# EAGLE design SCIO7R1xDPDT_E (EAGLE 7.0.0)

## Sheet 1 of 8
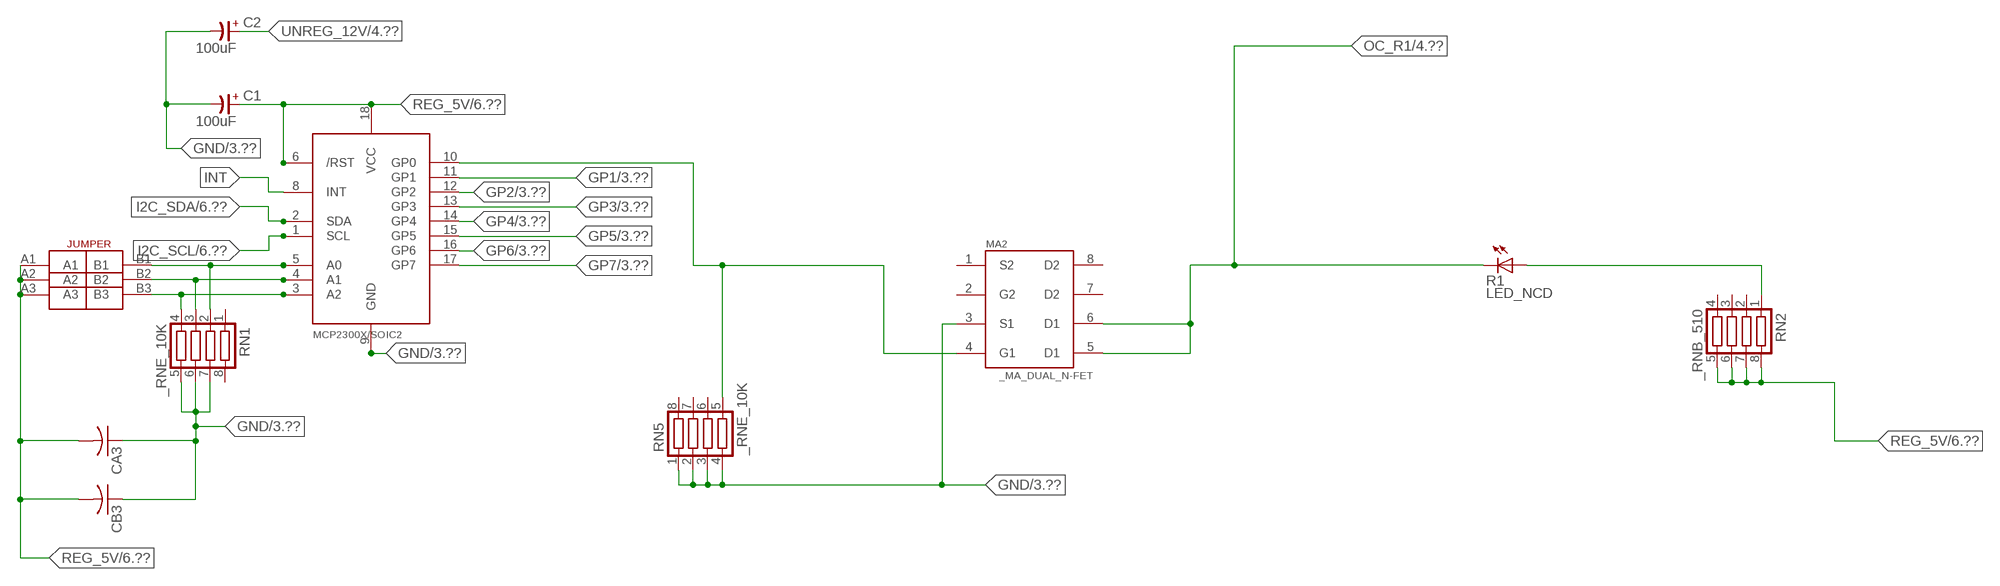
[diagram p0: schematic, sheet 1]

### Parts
C1  100uF  CP-E-025X060  [E-025X060]
C2  100uF  CP-E-025X060  [E-025X060]
CA3  CC1206KRX7R9BB104C1206K  [CC1206KRX7R9BB104]
CB3  TMK316F106ZL-TC1206K  [TMK316F106ZL-T]
IC2  MCP2300X/SO  [SO18W]
MA2  _MA_DUAL_N-FET  [_MA_DUAL_N-FET]
R1  LED_NCD  [CHIPLED_0603]
RN1  _RNE_10K  [RNE]
RN2  _RNB_510  [RNB]
RN5  _RNE_10K  [RNE]
U$18  JUMPER_3X2  [JUMPER_3X2]

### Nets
GND: C1.- C2.- CA3.1 CB3.1 IC2.9(GND) MA2.3(S1) RN1.5 RN1.6 RN1.7 RN5.1 RN5.2 RN5.3 RN5.4 ; also sheet 3,6,8
GP1: IC2.11(GP1) ; also sheet 3
GP2: IC2.12(GP2) ; also sheet 3
GP3: IC2.13(GP3) ; also sheet 3
GP4: IC2.14(GP4) ; also sheet 3
GP5: IC2.15(GP5) ; also sheet 3
GP6: IC2.16(GP6) ; also sheet 3
GP7: IC2.17(GP7) ; also sheet 3
I2C_SCL: IC2.1(SCL) ; also sheet 6
I2C_SDA: IC2.2(SDA) ; also sheet 6
INT: IC2.8(INT)
N$6: IC2.5(A0) RN1.2 U$18.B1
N$7: IC2.4(A1) RN1.3 U$18.B2
N$8: IC2.3(A2) RN1.4 U$18.B3
N$23: IC2.10(GP0) MA2.4(G1) RN5.5
N$32: R1.A RN2.1
OC_R1: MA2.5(D1) MA2.6(D1) R1.C ; also sheet 4
REG_5V: C1.+ CA3.2 CB3.2 IC2.6(/RST) IC2.18(VCC) RN2.5 RN2.6 RN2.7 RN2.8 U$18.A1 U$18.A2 U$18.A3 ; also sheet 6,8
UNREG_12V: C2.+ ; also sheet 4,6
Unconnected: MA2.2(G2) MA2.7(D2) MA2.8(D2) RN1.1 RN1.8 RN2.2 RN2.3 RN2.4 RN5.6 RN5.7 RN5.8

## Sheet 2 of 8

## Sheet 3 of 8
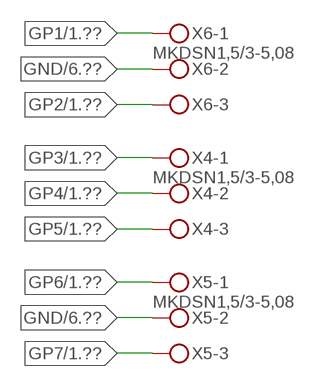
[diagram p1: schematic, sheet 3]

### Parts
X4  MKDSN1,5/3-5,08  [MKDSN1,5/3-5,08]
X5  MKDSN1,5/3-5,08  [MKDSN1,5/3-5,08]
X6  MKDSN1,5/3-5,08  [MKDSN1,5/3-5,08]

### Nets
GND: X5.2 X6.2 ; also sheet 1,6,8
GP1: X6.1 ; also sheet 1
GP2: X6.3 ; also sheet 1
GP3: X4.1 ; also sheet 1
GP4: X4.2 ; also sheet 1
GP5: X4.3 ; also sheet 1
GP6: X5.1 ; also sheet 1
GP7: X5.3 ; also sheet 1

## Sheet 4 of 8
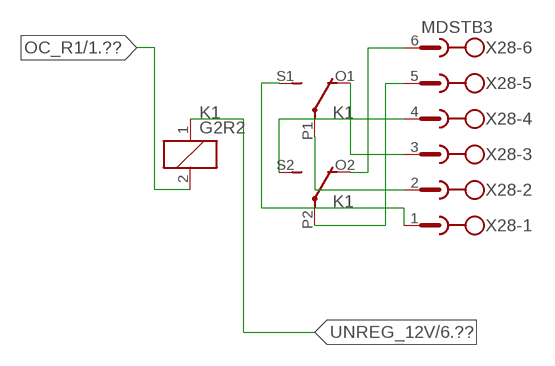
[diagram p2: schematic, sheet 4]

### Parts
K1  G2R2  [G2R2]
X28  MDSTB3  [MDSTB3]

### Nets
N$203: K1.P2(3:COM) X28.5
N$204: K1.O2(3:NC) X28.6
N$205: K1.S2(3:NO) X28.4
N$206: K1.P1(2:COM) X28.2
N$207: K1.O1(2:NC) X28.3
N$208: K1.S1(2:NO) X28.1
OC_R1: K1.2(1:C2) ; also sheet 1
UNREG_12V: K1.1(1:C1) ; also sheet 1,6

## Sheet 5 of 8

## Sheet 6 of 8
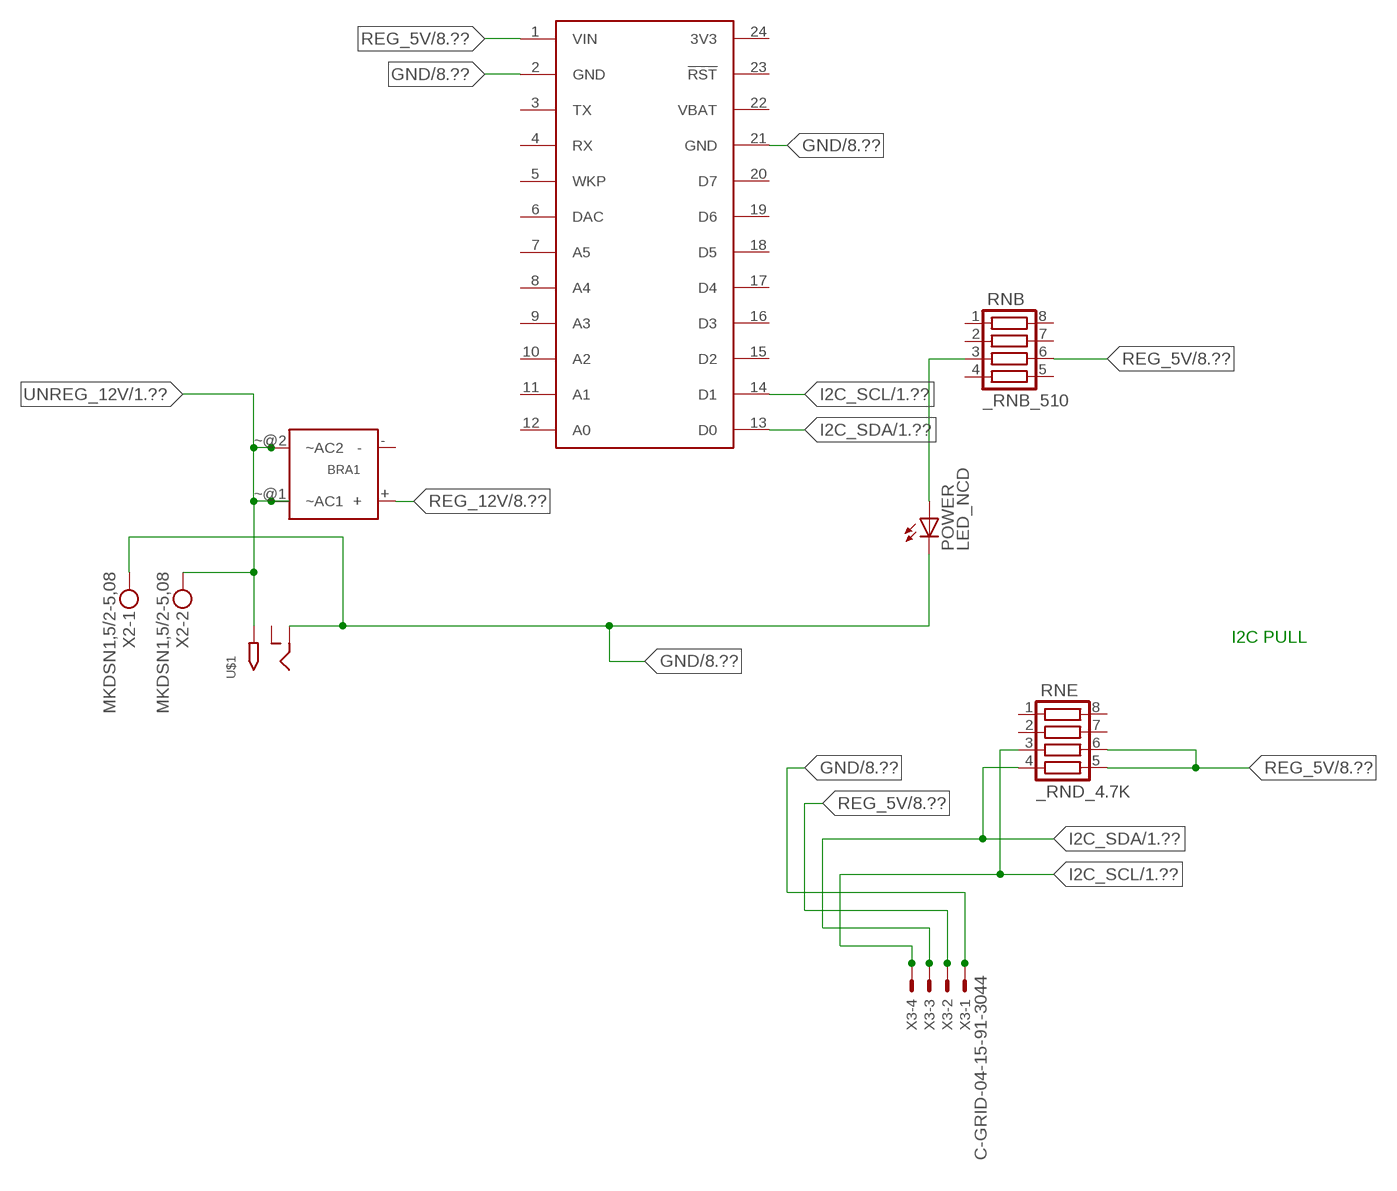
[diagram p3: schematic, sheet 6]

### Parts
BRA1  MB2S_  [MB2S]
POWER  LED_NCD  [CHIPLED_0603]
RNB  _RNB_510  [RNB]
RNE  _RND_4.7K  [RND]
S1  SPARK_CORECORE  [SPARK_CORE]
U$1  2.1MMJACK  [PJ-102A]
X2  MKDSN1,5/2-5,08  [MKDSN1,5/2-5,08]
X3  C-GRID-04-15-91-3044  [15-91-04]

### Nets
GND: POWER.C S1.2(GND) S1.21(GND) U$1.RING X2.1 X3.1 ; also sheet 1,3,8
I2C_SCL: RNE.3 S1.14(D1) X3.4 ; also sheet 1
I2C_SDA: RNE.4 S1.13(D0) X3.3 ; also sheet 1
N$2: POWER.A RNB.3
REG_5V: RNB.6 RNE.5 RNE.6 S1.1(VIN) X3.2 ; also sheet 1,8
REG_12V: BRA1.+ ; also sheet 8
UNREG_12V: BRA1.~@1(~AC1) BRA1.~@2(~AC2) U$1.TIP X2.2 ; also sheet 1,4
Unconnected: BRA1.- RNB.1 RNB.2 RNB.4 RNB.5 RNB.7 RNB.8 RNE.1 RNE.2 RNE.7 RNE.8 S1.3(TX) S1.4(RX) S1.5(WKP) S1.6(DAC) S1.7(A5) S1.8(A4) S1.9(A3) S1.10(A2) S1.11(A1) S1.12(A0) S1.15(D2) S1.16(D3) S1.17(D4) S1.18(D5) S1.19(D6) S1.20(D7) S1.23(!RST) U$1.RING_SW

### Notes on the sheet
- I2C PULL

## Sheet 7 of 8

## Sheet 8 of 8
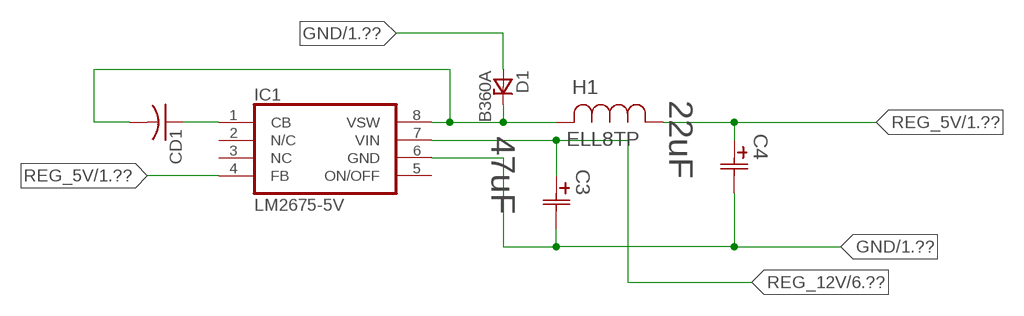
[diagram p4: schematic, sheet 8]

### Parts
C3  47uF  490-5463-6-NDCAP  [C2917(7343)-Y]
C4  22uF  490-5463-6-NDCAP  [C2917(7343)-Y]
CD1  _CD_10NF_50VC1206K  [_CD_10NF_50V]
D1  B360A  [DO214AC_ZENER]
H1  ELL8TP  [IND_ELL8TP]
IC1  LM2675-5V  LM2675  [SO-8]

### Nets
GND: C3.2(C2) C4.2(C2) D1.A IC1.6(GND) ; also sheet 1,3,6
N$1: CD1.2 D1.C H1.2 IC1.8(VSW)
N$3: CD1.1 IC1.1(CB)
REG_5V: C4.1(C1) H1.1 IC1.4(FB) ; also sheet 1,6
REG_12V: C3.1(C1) IC1.7(VIN) ; also sheet 6
Unconnected: IC1.2(N/C) IC1.5(ON/OFF)

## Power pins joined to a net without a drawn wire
3V3: S1.24(3V3)
NC: IC1.3(NC)
S2: MA2.1(S2)
VBAT: S1.22(VBAT)

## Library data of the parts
BRA1 = NCD_ULTIMATE_LIBRARY:MB2S: Bridge Rectifier BRA MB2S 200V 500ma Digikey MB2S-TPMSTR-ND/MB2S-TP
C1 C2 = NCD_ULTIMATE_LIBRARY:CP-: Capacitors All Kinds POLARIZED CAP
C3 C4 = NCD_ULTIMATE_bhaskar:490-5463-6-ND: NCD CAP
CA3 = NCD_ULTIMATE_LIBRARY:CC1206KRX7R9BB104: Capacitor CA .1uF 50V SMT C1206K CC1206KRX7R9BB104
CB3 = NCD_ULTIMATE_LIBRARY:TMK316F106ZL-T: Capacitor CB 10uF SMT 1206 TMK316F106ZL-T
CD1 = NCD_ULTIMATE_LIBRARY:_CD_10NF_50V: Capacitor 10nF SMT
D1 = NCD_ULTIMATE_bhaskar:B360A: NCD DIODE B350A/B360A
H1 = NCD_ULTIMATE_bhaskar:ELL8TP: NCD coil
IC1 = NCD_ULTIMATE_bhaskar:LM2675: LM2675 NCD http://www.ti.com/lit/ds/symlink/lm2675.pdf
IC2 = NCD_ULTIMATE_LIBRARY:MCP2300X: Semiconductor Port Expander I/O 8-Bit I2C MCP23008 Inexpensive i2c i/o expander - 8 general purpose i/o pins with optional pullups
K1 = NCD_ULTIMATE_LIBRARY:G2R2: RELAY 2 x switch, Omron
MA2 = NCD_ULTIMATE_LIBRARY:_MA_DUAL_N-FET: FET Dual N-Channel 8-SOIC NMOSFET Digikey 785-1064-2-ND/AO4842
POWER = NCD_ULTIMATE_bhaskar:LED_NCD
R1 = NCD_ULTIMATE_LIBRARY:LED_NCD: LED Digikey 754-1132-2-ND/APT2012SRCPRV
RN1 RN5 = NCD_ULTIMATE_LIBRARY:_RNE_10K: Resistor Array RNE SMT 10K x 4 Single Resistor Source: http://www.ctscorp.com/components/Datasheets/CTSChipArrayDs.pdf Digikey 742C083103JPTR-ND/742C083103JP; OC_FARNELL: unknown; OC_NEWARK: unknown
RN2 RNB = NCD_ULTIMATE_LIBRARY:_RNB_510: Resistor Array RNB SMT 510 x 4 Single Resistor Source: http://www.ctscorp.com/components/Datasheets/CTSChipArrayDs.pdf Digikey 742C083511JPTR-ND/ 742C083511JP; OC_FARNELL: unknown; OC_NEWARK: unknown
RNE = NCD_ULTIMATE_LIBRARY:_RND_4.7K: Resistor Array RND SMT 4.7K x 4 Single Resistor Source: http://www.ctscorp.com/components/Datasheets/CTSChipArrayDs.pdf Digikey 742C083472JPTR-ND/742C083472JP; OC_FARNELL: unknown; OC_NEWARK: unknown
S1 = Spark:SPARK_CORE
U$1 = NCD_ULTIMATE_CONNECTORS:2.1MMJACK: 2.1mm x 5.5mm DC jack with internal switch. Digikey part #PJ-102A, 4UCON part #05537 By microbuilder.eu
U$18 = NCD_ULTIMATE_CONNECTORS:JUMPER_3X2
X2 = NCD_ULTIMATE_CONNECTORS:MKDSN1,5/2-5,08: MKDSN 1,5/ 2-5,08 Printklemme
X3 = NCD_ULTIMATE_CONNECTORS:C-GRID-04: CONNECTOR 4-Pos I2C wire to board 2.54 mm (0.100") pitch header Digikey WM1342-ND/0015912045; OC_FARNELL: unknown; OC_NEWARK: unknown
X4-X6 = NCD_ULTIMATE_CONNECTORS:MKDSN1,5/3-5,08: MKDSN 1,5/ 3-5,08 Printklemme Nennstrom: 13,5 A Nennspannung: 250 V Rastermaß: 5,08 mm Polzahl: 3 Anschlussart: Schraubanschluss Montage: Löten Anschlussrichtung Leiter/Platine: 0 ° Artikelnummer: 1729131 Source: http://eshop.phoenixcontact.com .. 1729131.pdf
X28 = NCD_ULTIMATE_LIBRARY:MDSTB3: PHOENIX

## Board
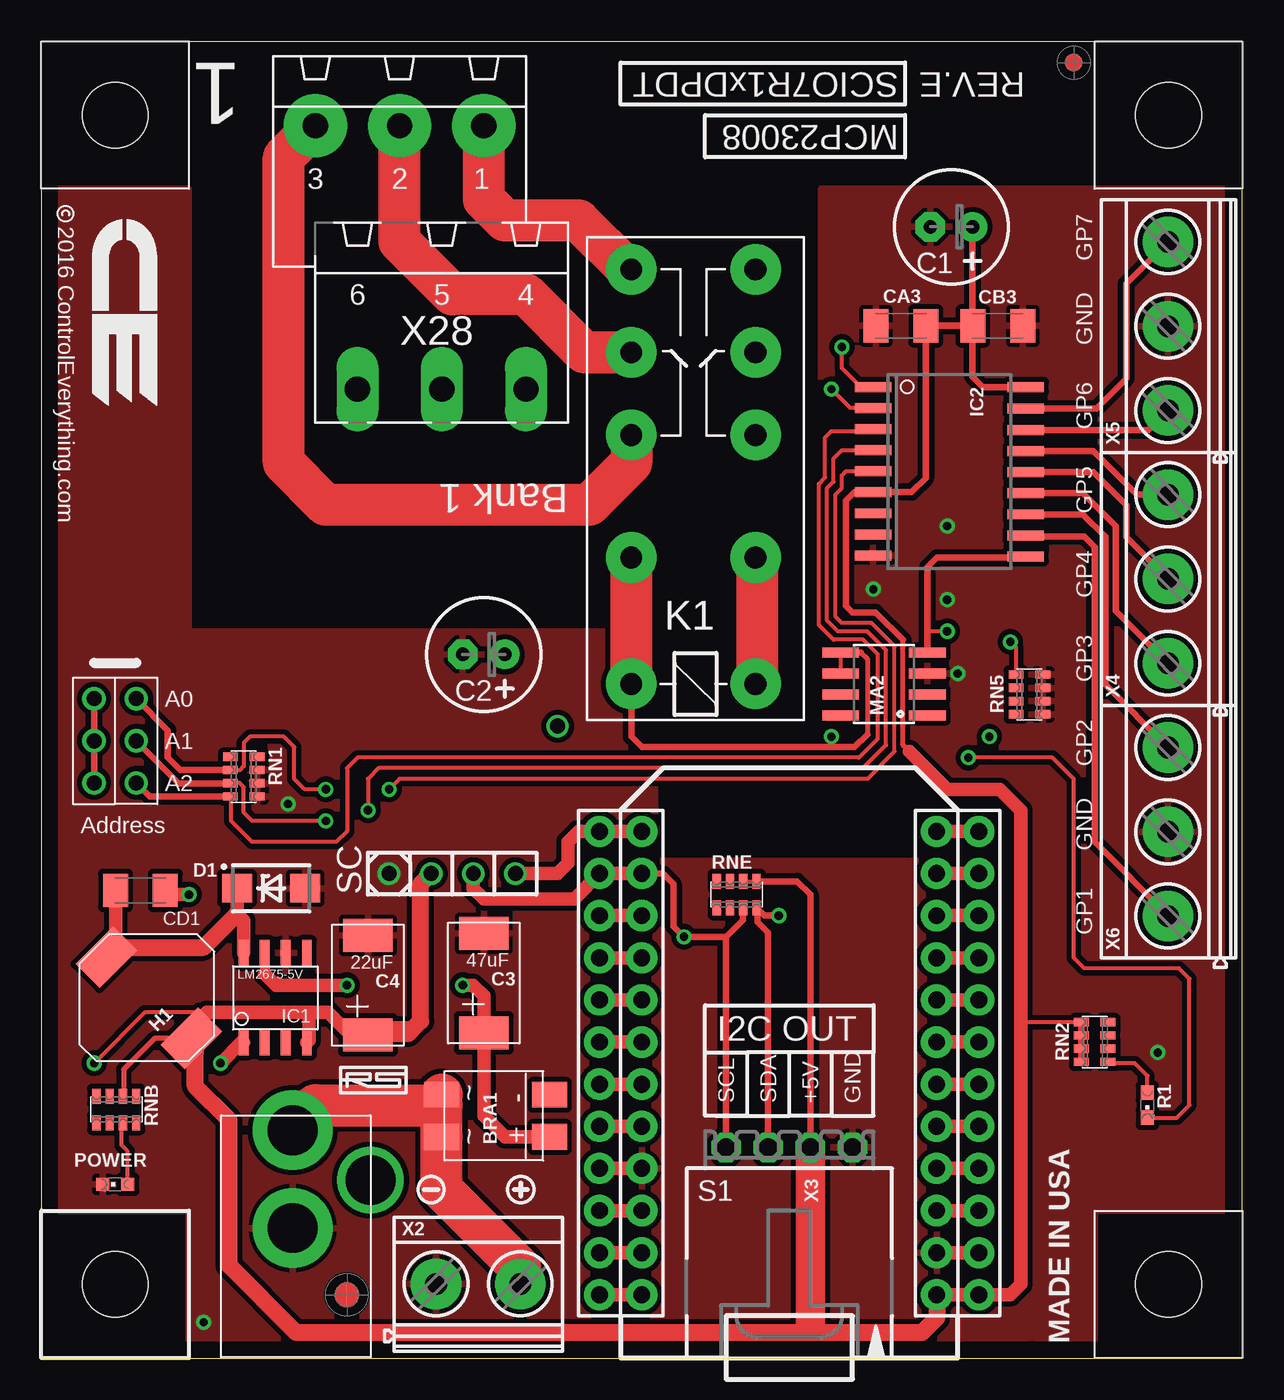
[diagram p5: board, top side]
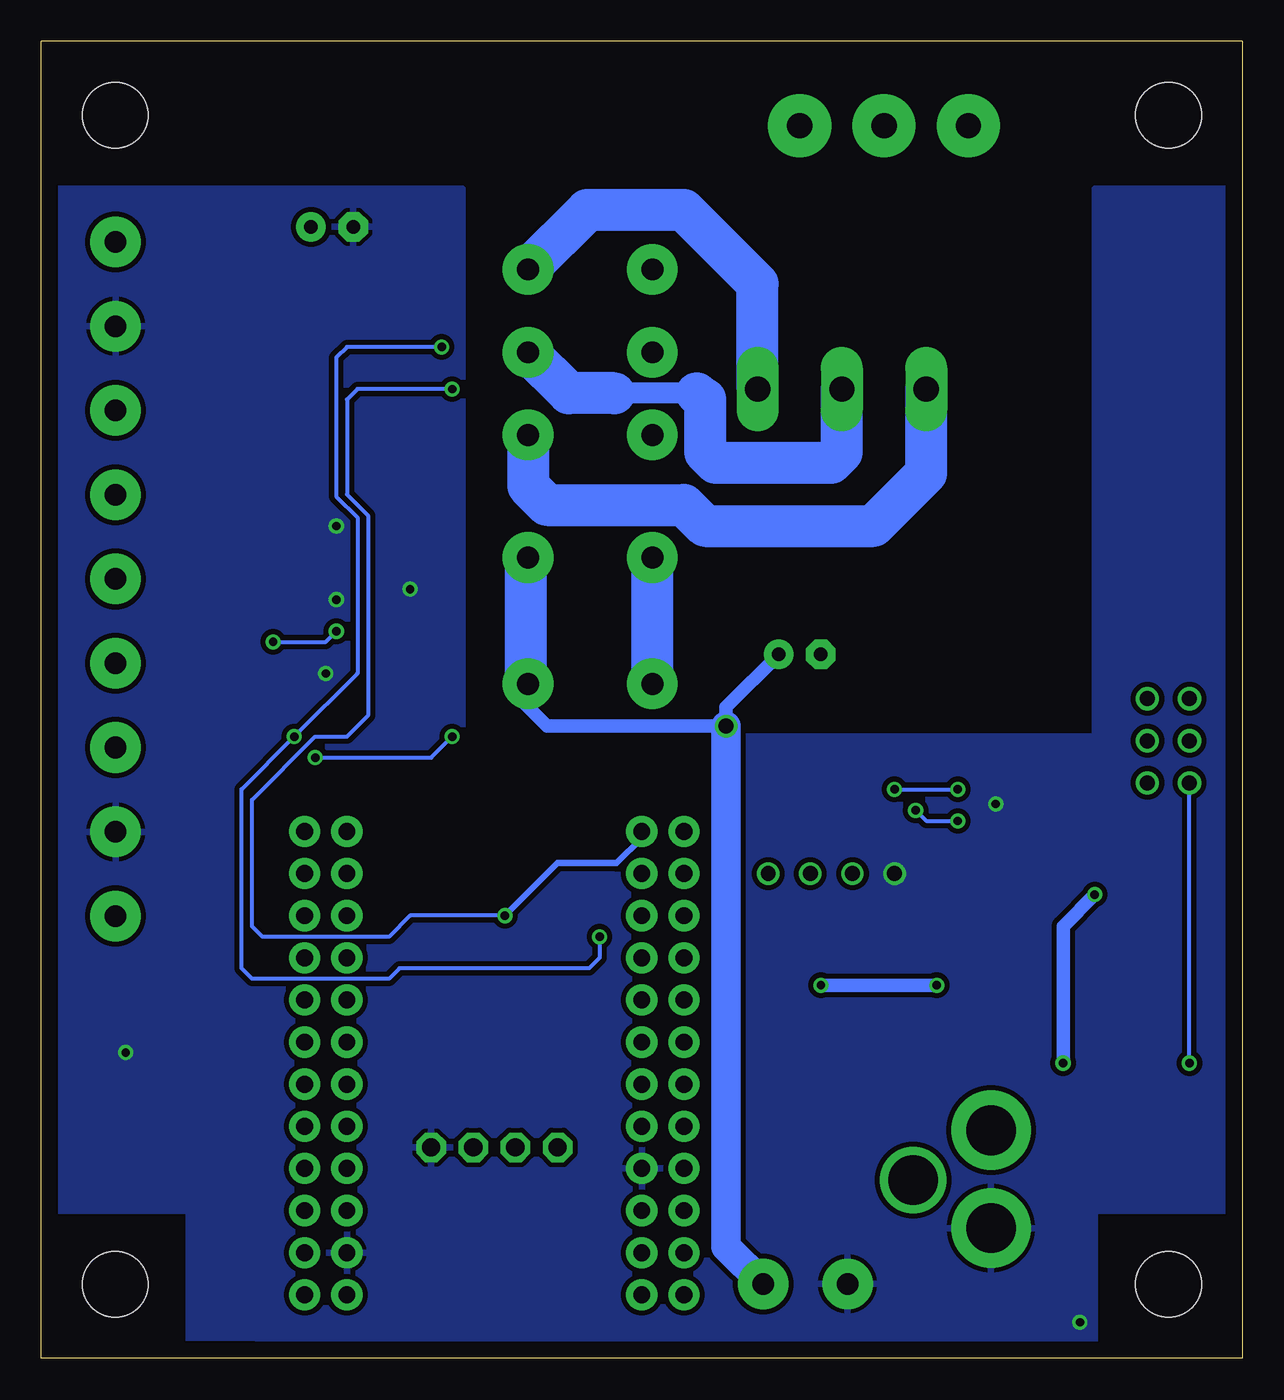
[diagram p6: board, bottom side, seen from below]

Size 72.39 x 79.38 mm. Coordinates in mm from the lower left corner, seen from the top.
Outline: 59.69,0 61.58,0
Outline: 59.69,0 72.39,0 72.39,79.38 0,79.38 0,0 59.69,0
Copper layers (1*16): Top 0.035mm / dielectric 1.5mm / Bottom 0.035mm
Design rules "default": minimum track width 10mil, minimum drill 24mil, track to track 8mil, track to pad 8mil, pad to pad 8mil, via to via 8mil, smd to smd 8mil, copper to edge 40mil, drill to drill 8mil, minimum pad ring 10mil, minimum via ring 8mil, stop-mask expansion 4mil, vias tented up to drill 0mil, thermal gap 10mil
Holes 3.96 mm at 4.45,4.45 4.45,4.45

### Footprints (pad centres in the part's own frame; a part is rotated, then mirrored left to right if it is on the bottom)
MB2S = smd 1.55 x 2.1: + 0,-6.5; - 2.54,-6.5; ~@1 0,0; ~@2 2.54,0
E-025X060 = drill 0.813 pad 1.778: + -1.27,0 | drill 0.813 pad 1.778 octagon: - 1.27,0
C2917(7343)-Y = smd 2 x 3: 1 -3,0; 2 3,0
CC1206KRX7R9BB104 = smd 1.5 x 2: 1 -1.5,0; 2 1.5,0
TMK316F106ZL-T = smd 1.5 x 2: 1 -1.5,0; 2 1.5,0
_CD_10NF_50V = smd 1.5 x 2: 1 -1.5,0; 2 1.5,0
DO214AC_ZENER = smd 1.8 x 1.7: A 2.05,0; C -2.05,0
IND_ELL8TP = smd 2.054 x 3.2 rotated 45: 1 -2.442,-2.696; 2 2.442,2.442
SO-8 = smd 0.6 x 1.55: 1 -1.905,-2.69; 2 -0.635,-2.69; 3 0.635,-2.69; 4 1.905,-2.69; 5 1.905,2.71; 6 0.635,2.71; 7 -0.635,2.71; 8 -1.905,2.71
SO18W = smd 0.6 x 2.2: 1 -4.445,-4.6; 2 -3.175,-4.6; 3 -1.905,-4.6; 4 -0.635,-4.6; 5 0.635,-4.6; 6 1.905,-4.6; 7 3.175,-4.6; 8 4.445,-4.6; 9 5.715,-4.6; 10 5.775,4.6; 11 4.505,4.6; 12 3.235,4.6; 13 1.965,4.6; 14 0.695,4.6; 15 -0.575,4.6; 16 -1.845,4.6; 17 -3.145,4.6; 18 -4.445,4.6
G2R2 = drill 1.321 pad 3.048: 1 -2.54,-3.683; 2 -2.54,3.81; 3 5.08,-3.683; 4 5.08,3.81; O1 12.471,3.81; O2 12.471,-3.683; P1 17.45,3.81; P2 17.45,-3.683; S1 22.454,3.81; S2 22.454,-3.683
_MA_DUAL_N-FET = smd 0.61 x 2.21: 1 -1.905,-2.616; 2 -0.635,-2.616; 3 0.635,-2.616; 4 1.905,-2.616; 5 1.905,2.616; 6 0.635,2.616; 7 -0.635,2.616; 8 -1.905,2.616
CHIPLED_0603 = smd 0.8 x 0.8: A 0,-0.75; C 0,0.75
CHIPLED_0603' = smd 0.8 x 0.876: A 0,-0.75; C 0,0.75
RNE = smd 0.5 x 0.9: 1 -1.2,-0.8; 2 -0.4,-0.8; 3 0.4,-0.8; 4 1.2,-0.8; 5 1.2,0.8; 6 0.4,0.8; 7 -0.4,0.8; 8 -1.2,0.8
RNB = smd 0.5 x 0.9: 1 -1.2,-0.8; 2 -0.4,-0.8; 3 0.4,-0.8; 4 1.2,-0.8; 5 1.2,0.8; 6 0.4,0.8; 7 -0.4,0.8; 8 -1.2,0.8
RND = smd 0.5 x 0.9: 1 -1.2,-0.8; 2 -0.4,-0.8; 3 0.4,-0.8; 4 1.2,-0.8; 5 1.2,0.8; 6 0.4,0.8; 7 -0.4,0.8; 8 -1.2,0.8
SPARK_CORE = drill 1.016 pad 1.88: 1 -8.89,13.97; 2 -8.89,11.43; 3 -8.89,8.89; 4 -8.89,6.35; 5 -8.89,3.81; 6 -8.89,1.27; 7 -8.89,-1.27; 8 -8.89,-3.81; 9 -8.89,-6.35; 10 -8.89,-8.89; 11 -8.89,-11.43; 12 -8.89,-13.97; 13 8.89,-13.97; 14 8.89,-11.43; 15 8.89,-8.89; 16 8.89,-6.35; 17 8.89,-3.81; 18 8.89,-1.27; 19 8.89,1.27; 20 8.89,3.81; 21 8.89,6.35; 22 8.89,8.89; 23 8.89,11.43; 24 8.89,13.97; 25 -11.43,13.97; 26 -11.43,11.43; 27 -11.43,8.89; 28 -11.43,6.35; 29 -11.43,3.81; 30 -11.43,1.27; 31 -11.43,-1.27; 32 -11.43,-3.81; 33 -11.43,-6.35; 34 -11.43,-8.89; 35 -11.43,-11.43; 36 -11.43,-13.97; 37 11.43,13.97; 38 11.43,11.43; 39 11.43,8.89; 40 11.43,6.35; 41 11.43,3.81; 42 11.43,1.27; 43 11.43,-1.27; 44 11.43,-3.81; 45 11.43,-6.35; 46 11.43,-8.89; 47 11.43,-11.43; 48 11.43,-13.97
PJ-102A = drill 3 pad 4.8: RING 0.1,-3.39; TIP 0.1,-9.29 | drill 3 pad 3.251: RING_SW -4.6,-6.29
PCB_MOUNTING_HOLE = hole 3.962: 4.445,4.445
JUMPER_3X2 = drill 0.9: A1 0,5.08; A2 0,2.54; A3 0,0; B1 2.54,5.08; B2 2.54,2.54; B3 2.54,0
MKDSN1,5/2-5,08 = drill 1.3 pad 3.048: 1 -2.561,0.025; 2 2.519,0.025
15-91-04 = drill 1.1 pad 1.778 octagon: 1 -3.81,-7.62; 2 -1.27,-7.62; 3 1.27,-7.62; 4 3.81,-7.62
MKDSN1,5/3-5,08 = drill 1.3 pad 3.048: 1 -7.641,0.025; 2 -2.561,0.025; 3 2.519,0.025
MDSTB3 = drill 1.524 pad 3.81: 1 -3.81,-10.795; 2 1.27,-10.795; 3 6.35,-10.795 | drill 1.524 pad 2.54 long: 4 -6.35,5.08; 5 -1.27,5.08; 6 3.81,5.08

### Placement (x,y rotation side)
BRA1  24.13,13.34 90 top
C1  54.86,68.2 180 top
C2  26.67,42.42 180 top
C3  26.67,22.61 90 top
C4  19.68,22.48 90 top
CA3  51.82,62.23 0 top
CB3  57.66,62.23 180 top
CD1  5.97,28.19 180 top
D1  13.84,28.32 0 top
H1  6.35,21.72 90 top
IC1  14.1,21.72 0 top
IC2  54.74,54.1 270 top
K1  39.37,43.18 90 top
MA2  50.8,40.64 90 top
POWER  4.45,10.48 90 top
R1  LED_NCD  [CHIPLED_0603']  66.67,15.24 180 top
RN1  12.19,35.05 270 top
RN2  63.5,19.05 90 top
RN5  59.56,40 90 top
RNB  4.51,14.99 0 top
RNE  41.91,27.94 0 top
S1  45.09,17.78 180 top
U$1  15.24,4.45 180 top
U$4  PCB_MOUNTING_HOLE  [PCB_MOUNTING_HOLE]  72.39,70.48 90 top
U$6  PCB_MOUNTING_HOLE  [PCB_MOUNTING_HOLE]  72.39,0 90 top
U$7  PCB_MOUNTING_HOLE  [PCB_MOUNTING_HOLE]  8.89,70.48 90 top
U$10  [VISION_REF15]  18.41,3.81 0 top
U$18  3.17,34.67 0 top
U$19  [VISION_REF10]  62.23,78.11 0 top
U$21  [ICON_USA]  61.98,0.89 90 top
U$22  [ICON_MINUS]  23.5,10.16 180 top
U$24  [ICON_PLUS]  28.89,10.16 90 top
X2  26.35,4.45 0 top
X3  45.09,5.08 180 top
X4  67.94,49.53 90 top
X5  67.94,64.77 90 top
X6  67.94,34.29 90 top
X28  22.86,63.5 180 top

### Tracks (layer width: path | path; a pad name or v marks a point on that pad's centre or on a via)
GND  (via drill 0.5, 0.9)
  other vias: 14.86,33.4 54.61,45.72 54.61,50.16 67.31,18.41 50.16,46.35 55.24,41.27 9.78,2.16 20.95,29.21
  pour Bottom (isolate 0.305): -2.54,8.89 8.89,8.89 8.89,0 63.5,0 63.5,8.89 71.75,8.89 71.75,70.48 46.99,70.48 46.99,37.46 8.89,37.46 8.89,70.48 -2.54,70.48
  pour Top (isolate 0.305): -4.45,8.89 8.89,8.89 8.89,0 63.5,0 63.5,8.89 71.75,8.89 71.75,70.48 46.99,70.48 46.99,43.81 8.89,43.81 8.89,70.48 -4.45,70.48
GP1
  Top 0.406: X6.1 67.92,26.7 63.5,31.12 63.5,48.89 62.87,49.53 59.4,49.53 IC2.11
GP2
  Top 0.406: IC2.12 62.8,50.87 64.14,49.53 64.14,40.59 X6.3
GP3
  Top 0.406: IC2.13 62.8,52.14 64.77,50.16 64.77,45.04 X4.1
GP4
  Top 0.406: IC2.14 63.43,53.41 65.41,51.43 65.41,49.48 X4.2
GP5
  Top 0.406: IC2.15 63.43,54.68 66.04,52.07 67.9,52.07 X4.3
GP6
  Top 0.406: IC2.16 66.74,55.95 X5.1
GP7
  Top 0.406: IC2.17 63.6,57.25 65.41,59.05 65.41,64.77 X5.3
I2C_SCL  (via drill 0.5, 0.9)
  Top 0.254: IC2.1 49.4,58.55 48.26,59.69 v48.26,60.96
  Top 0.406: X3.4 41.27,25.4 | 41.27,25.4 42.29,26.42 42.29,27.12 RNE.3 | S1.14 37.47,29.21 38.1,28.57 38.1,26.04 v38.73,25.4 41.27,25.4
  Top 0.813: v26.04,29.21 26.04,28.32 26.67,27.69 32.13,27.69 33.66,29.21
  Bottom 0.254: v48.26,60.96 53.98,60.96 54.61,60.32 54.61,51.94 53.34,50.67 53.34,41.27 v57.15,37.46 60.33,34.29 60.33,23.5 59.69,22.86 51.44,22.86 50.8,23.5 39.37,23.5 38.73,24.13 v38.73,25.4
I2C_SDA  (via drill 0.5, 0.9)
  Top 0.254: IC2.2 48.77,57.28 v47.62,58.42
  Top 0.406: X3.3 43.81,25.65 43.18,26.29 43.18,27.07 RNE.4 43.58,26.67 v44.45,26.67
  Top 0.813: v28.57,29.21 31.11,29.21 31.75,29.85 31.75,31.12 32.38,31.75 33.66,31.75
  Bottom 0.254: v47.62,58.42 53.34,58.42 53.98,57.78 53.98,52.07 52.7,50.8 52.7,38.73 53.98,37.46 55.88,37.46 59.69,33.66 59.69,26.04 59.05,25.4 51.44,25.4 50.16,26.67 v44.45,26.67
  Bottom 0.406: S1.13 36.2,31.37 37.72,29.85 41.27,29.85 v44.45,26.67
N$1
  Top 0.813: H1.2 3.88,24.77 | D1.C 11.79,26.78 12.19,26.38 IC1.8 | CD1.2 4.47,24.79 4.45,24.77
  Top 1.016: 3.88,24.77 4.45,24.77 9.78,24.77 11.79,26.78
N$2
  Top 0.254: POWER.A 5.2,12.46 4.83,12.83 4.83,14.1 RNB.3
  Top 0.406: 4.95,14.14 RNB.3
N$3  (via drill 0.5)
  Top 0.813: IC1.1 12.04,19.03 v10.79,17.78 | v8.89,27.94 7.72,27.94 CD1.1
  Bottom 0.813: v10.79,17.78 10.79,26.04 v8.89,27.94
N$6  (via drill 0.5)
  Top 0.254: v20.95,34.29 21.59,34.92 49.78,34.92 51.44,36.58 51.44,42.93 50.04,44.32 48.26,44.32 47.88,44.7 47.88,52.07 48.26,52.45 48.26,53.21 48.51,53.47 IC2.5 50.01,53.34 | v17.14,34.29 15.88,34.29 15.24,34.92 15.24,36.83 14.61,37.46 12.57,37.46 12.19,37.08 12.19,35.69 11.94,35.43 11.41,35.43 RN1.2
  Top 0.406: RN1.2 8.36,35.45 7.62,36.2 7.62,37.85 U$18.B1
  Bottom 0.254: v20.95,34.29 v17.14,34.29
N$7  (via drill 0.5)
  Top 0.254: v19.68,33.02 19.68,34.92 20.32,35.56 49.53,35.56 50.93,36.96 50.93,42.67 49.78,43.81 48.01,43.81 47.37,44.45 47.37,52.45 47.75,52.83 47.75,54.23 48.26,54.74 IC2.4 50.01,54.61 | v17.14,32.38 12.7,32.38 12.19,32.89 12.19,34.42 11.94,34.67 11.41,34.67 RN1.3
  Top 0.406: RN1.3 8.27,34.65 U$18.B2
  Bottom 0.254: v19.68,33.02 19.05,32.38 v17.14,32.38
N$8
  Top 0.254: RN1.4 11.43,33.81 11.43,32.38 12.7,31.12 17.78,31.12 18.41,31.75 18.41,35.56 19.05,36.2 49.28,36.2 50.42,37.34 50.42,42.42 49.53,43.31 47.75,43.31 46.86,44.2 46.86,52.7 47.24,53.09 47.24,55.5 47.62,55.88 50.01,55.88 IC2.3
  Top 0.406: RN1.4 6.53,33.85 U$18.B3
N$23  (via drill 0.5)
  Top 0.254: RN5.5 58.76,42.84 v58.42,43.18 | v54.61,43.81 53.42,43.81
  Top 0.406: MA2.4 53.42,43.81 53.42,47.7 53.98,48.26 59.27,48.26 IC2.10
  Bottom 0.254: v58.42,43.18 55.24,43.18 v54.61,43.81
N$32
  Top 0.254: R1.A 66.67,17.02 65.91,17.78 64.37,17.78 RN2.1
N$203
  Bottom 1.27: 32.89,58.17 37.85,58.17
  Bottom 2.54: 24.13,57.15 X28.5 24.13,54.61 24.77,53.97 31.75,53.97 32.38,54.61 32.38,57.78 32.89,58.17 | 37.85,58.17 40.59,58.17 K1.P2
N$204
  Bottom 2.54: K1.O2 43.05,52.58 41.91,51.43 33.66,51.43 32.38,50.16 22.23,50.16 19.05,53.34 X28.6
N$205
  Bottom 2.54: X28.4 29.21,64.77 33.66,69.22 39.47,69.22 K1.S2
N$206
  Top 2.54: K1.P1 32.72,60.63 29.21,64.14 24.77,64.14 21.59,67.31 X28.2
N$207
  Top 2.54: K1.O1 35.56,53.97 33.02,51.43 17.14,51.43 14.61,53.97 14.61,72.39 X28.3
N$208
  Top 2.54: K1.S1 35.33,65.63 32.38,68.58 27.94,68.58 26.67,69.85 X28.1
OC_R1  (via drill 0.5)
  Top 0.254: MA2.5 MA2.6 | R1.C 68.47,14.49 69.22,15.24 69.22,22.86 68.58,23.5 62.87,23.5 62.23,24.13 62.23,34.92 60.96,36.2 v55.88,36.2 | v47.62,37.46 47.62,36.83
  Top 0.305: 49.4,42.54 49.78,42.16 49.78,37.59
  Top 0.406: MA2.5 49.4,42.54 | 49.78,37.59 49.02,36.83 47.62,36.83 36.2,36.83 35.56,37.46 K1.2
  Bottom 0.254: v55.88,36.2 48.9,36.2 v47.62,37.46
REG_5V  (via drill 0.5, 0.9)
  Top 0.254: RNE.6 RNE.5 | RN2.5 59.12,20.25 59.05,20.32 | 9.96,20.83 6.22,20.83 v3.17,17.78
  Top 0.305: 51.94,43.31 51.94,36.96 52.32,36.58 | H1.1 6.83,19.28 4.95,17.4 4.95,15.83 RNB.6
  Top 0.406: U$18.A3 U$18.A2 U$18.A1 | RN2.8 RN2.7 RN2.6 RN2.5 | 51.94,43.31 50.29,44.96 48.9,44.96 48.51,45.34 48.51,51.69 49.02,52.2 IC2.6 52.45,52.2 53.32,53.06 CA3.2 CB3.2 56.13,62.21 | IC2.18 56.77,58.55 56.13,59.18 56.13,62.21 | C1.+ 56.13,62.21 | RNE.5 45.55,28.74 46.35,27.94 X3.2
  Top 0.813: 16.13,20.83 9.96,20.83 H1.1 | 16.13,20.83 17.27,20.83 18.41,19.69 20.75,19.69 C4.1 | IC1.4 16.13,19.15 16.13,20.83 | 56.52,3.81 58.42,3.81 59.05,4.45 59.05,20.32 59.05,33.02 57.78,34.29 54.61,34.29 52.32,36.58
  Top 1.016: 46.35,2.16 46.35,1.52 | 46.35,1.52 15.37,1.52 11.3,5.59 11.3,14.35 9.27,16.38 9.27,18.41 H1.1 | 22.05,19.69 22.23,19.69 22.86,20.32 22.86,28.57 v23.5,29.21 | S1.1 53.98,2.41 53.09,1.52 46.35,1.52
  Top 1.27: 20.75,19.69 22.05,19.69
  Top 1.778: X3.2 46.35,2.16
  Bottom 0.254: v3.17,17.78 U$18.A3
REG_12V  (via drill 0.5)
  Top 0.61: IC1.7 13.46,23.16 | 14.1,22.48 14.15,22.48
  Top 0.813: v18.41,22.48 14.15,22.48 13.46,23.16 | v25.4,22.48 26.04,22.48 26.67,21.84 C3.1 26.67,14.61 27.94,13.34 BRA1.+
  Bottom 0.813: v18.41,22.48 v25.4,22.48
UNREG_12V  (via drill 0.9)
  Top 2.54: X2.2 28.87,5.42 24.13,10.16 BRA1.~@1 24.13,15.24 | 24.13,15.24 BRA1.~@2 | U$1.TIP 15.14,13.87 16.51,15.24 24.13,15.24
  Bottom 0.813: K1.1 43.18,40.51 43.18,39.37 41.91,38.1 v31.11,38.1 31.11,39.24 C2.+
  Bottom 1.778: v31.11,38.1 31.11,6.71 X2.2

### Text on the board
tNames: 1 | SCIO7R1xDPDT | REV.E | MCP23008 | 2016 ControlEverything.com | GP7 | GND | GP6 | Bank 1 | GP5 | GP4 | GP3 | A0 | A1 | GP2 | A2 | Address | GND | SC | GP1 | I2C OUT | SCL | SDA | +5V | GND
